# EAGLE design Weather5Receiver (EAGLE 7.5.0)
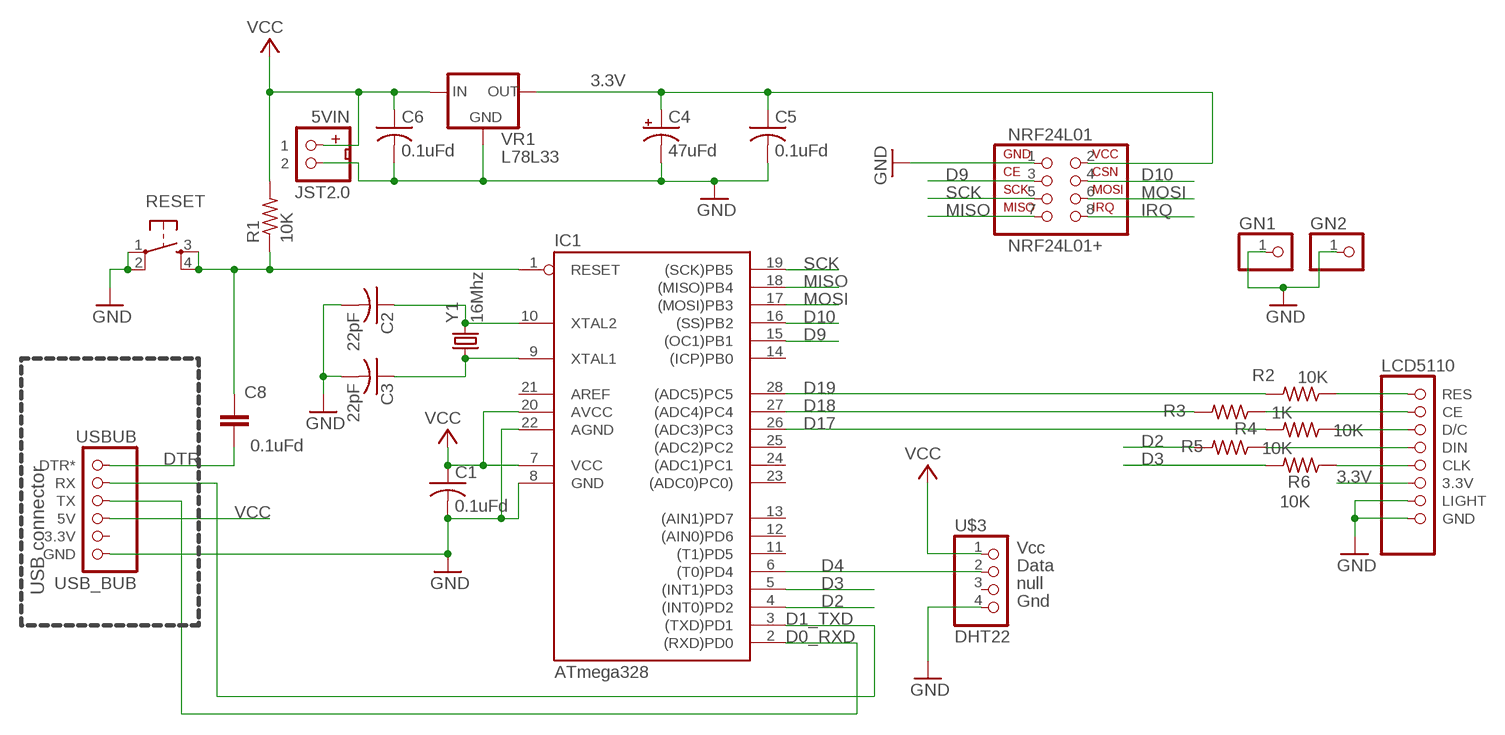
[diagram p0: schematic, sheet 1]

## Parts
5VIN  JST2.0  [JST2.0]
C1  0.1uFd  C-US050-025X075  [C050-025X075]
C2  22pF  C-US025-025X050  [C025-025X050]
C3  22pF  C-US025-025X050  [C025-025X050]
C4  47uFd  CPOL-USE2,5-6E  [E2,5-6E]
C5  0.1uFd  C-US025-025X050  [C025-025X050]
C6  0.1uFd  C-US025-025X050  [C025-025X050]
C8  0.1uFd  C-EU050-025X075  [C050-025X075]
GN1  PINHD-1X1  [1X01]
GN2  PINHD-1X1  [1X01]
IC1  ATmega328  AT90S4433P  [DIL28-3]
LCD5110  LCD5110_1TOP  [LCD5110T1]
NRF24L01  NRF24L01+  [NRF24L01+]
R1  10K  R-US_0207/2V  [0207/2V]
R2  10K  R-US_0207/5V  [0207/5V]
R3  1K  R-US_0207/5V  [0207/5V]
R4  10K  R-US_0207/5V  [0207/5V]
R5  10K  R-US_0207/5V  [0207/5V]
R6  10K  R-US_0207/5V  [0207/5V]
RESET  TAC_SWITCHPTH  [TACTILE-PTH]
U$3  DHT22  [1X04]
USBUB  USB_BUB  [USB_BUB]
VR1  L78L33  78LXX  [78LXX]
Y1  16Mhz  CRYSTALHC49US  [HC49US]

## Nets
3.3V: C4.+ C5.1 LCD5110.3.3V NRF24L01.2 VR1.OUT
D0_RXD: IC1.2((RXD)PD0) USBUB.TX
D1_TXD: IC1.3((TXD)PD1) USBUB.RX
D2: IC1.4((INT0)PD2) R5.2
D3: IC1.5((INT1)PD3) R6.2
D4: IC1.6((T0)PD4) U$3.2(DATA)
D9: IC1.15((OC1)PB1) NRF24L01.3
D10: IC1.16((SS)PB2) NRF24L01.4
D17: IC1.26((ADC3)PC3) R4.2
D18: IC1.27((ADC4)PC4) R3.2
D19: IC1.28((ADC5)PC5) R2.2
DTR: C8.1 USBUB.DTR*
GND [power]: 5VIN.2 C1.2 C2.2 C3.2 C4.- C5.2 C6.2 GN1.1 GN2.1 IC1.8(GND) IC1.22(AGND) LCD5110.GND LCD5110.LIGHT NRF24L01.1 RESET.1 RESET.2 U$3.4(GND) USBUB.GND VR1.GND
IRQ: NRF24L01.8
MISO: IC1.18((MISO)PB4) NRF24L01.7
MOSI: IC1.17((MOSI)PB3) NRF24L01.6
N$1: LCD5110.RES R2.1
N$3: LCD5110.CE R3.1
N$5: LCD5110.D/C R4.1
N$6: C3.1 IC1.9(XTAL1) Y1.1
N$7: C2.1 IC1.10(XTAL2) Y1.2
N$8: LCD5110.DIN R5.1
N$9: LCD5110.CLK R6.1
RESET: C8.2 IC1.1(RESET) R1.1 RESET.3 RESET.4
SCK: IC1.19((SCK)PB5) NRF24L01.5
VCC: 5VIN.1 C1.1 C6.1 IC1.7(VCC) IC1.20(AVCC) R1.2 U$3.1(VCC) USBUB.5V VR1.IN
Unconnected: IC1.11((T1)PD5) IC1.12((AIN0)PD6) IC1.13((AIN1)PD7) IC1.14((ICP)PB0) IC1.21(AREF) IC1.23((ADC0)PC0)) IC1.24((ADC1)PC1) IC1.25((ADC2)PC2) U$3.3(NULL) USBUB.3.3V

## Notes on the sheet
- USB connector

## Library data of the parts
5VIN = MTS_Custom:JST2.0: JST 2.0 2 pin connector 2mm spacing
C1-C3 C5 C6 = MTS:C-US: CAPACITOR, American symbol
C4 = rcl:CPOL-US: POLARIZED CAPACITOR, American symbol
C8 = my-rcl:C-EU: CAPACITOR, European symbol
GN1 GN2 = pinhead:PINHD-1X1: PIN HEADER
IC1 = atmel:AT90S4433: MICROCONTROLLER 4 Kbytes FLASH 128 bytes SRAM 256 bytes EEPROM UART 6-channel 10 bit ADC
LCD5110 = MTS_Custom:LCD5110_1
NRF24L01 = MTS_Custom:NRF24L01+: 2.4GHz Transceiver
R1-R6 = MTS:R-US_: RESISTOR, American symbol
RESET = SparkFun:TAC_SWITCH: Momentary Switch Button commonly used for reset or general input. Spark Fun Electronics SKU : COM-00097
U$3 = MTS_Custom:DHT22: This is a Temperature RH sensor. AKA AMM2303
USBUB = MTS:USB_BUB
VR1 = v-reg:78LXX: VOLTAGE REGULATOR
Y1 = MTS:CRYSTAL: Crystals

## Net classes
0 default: width 0.4 mm, clearance 0.3 mm
1 power: width 0.6 mm, clearance 0.3 mm

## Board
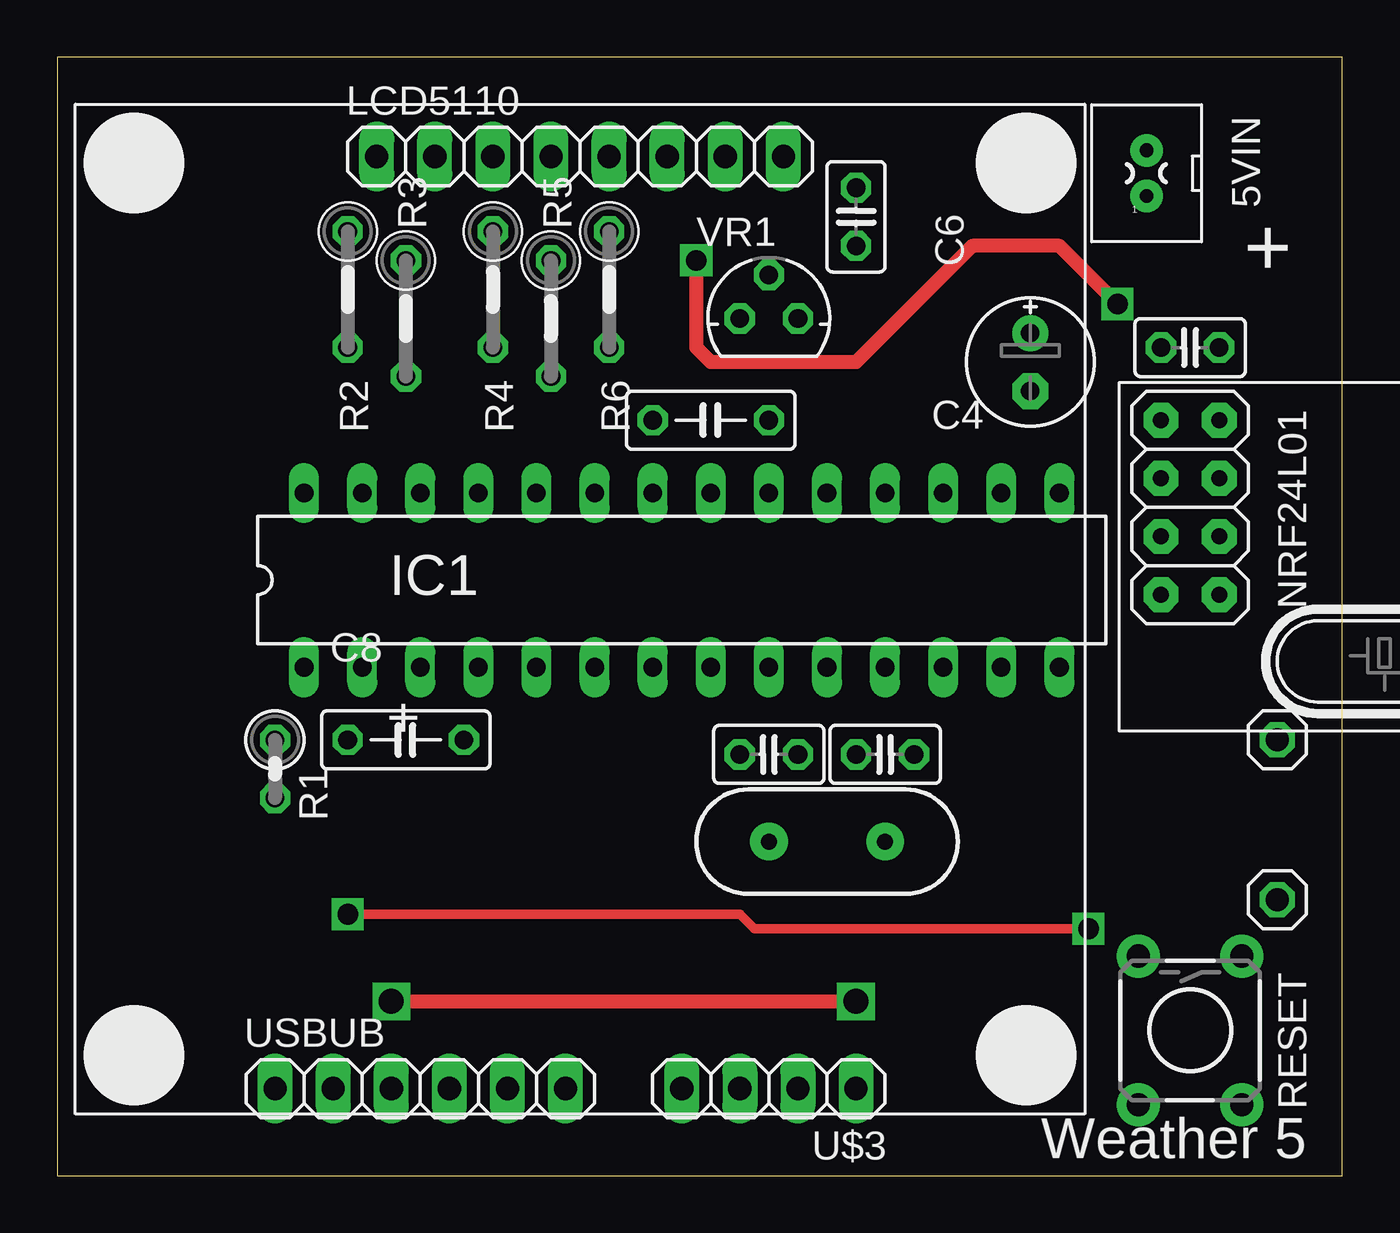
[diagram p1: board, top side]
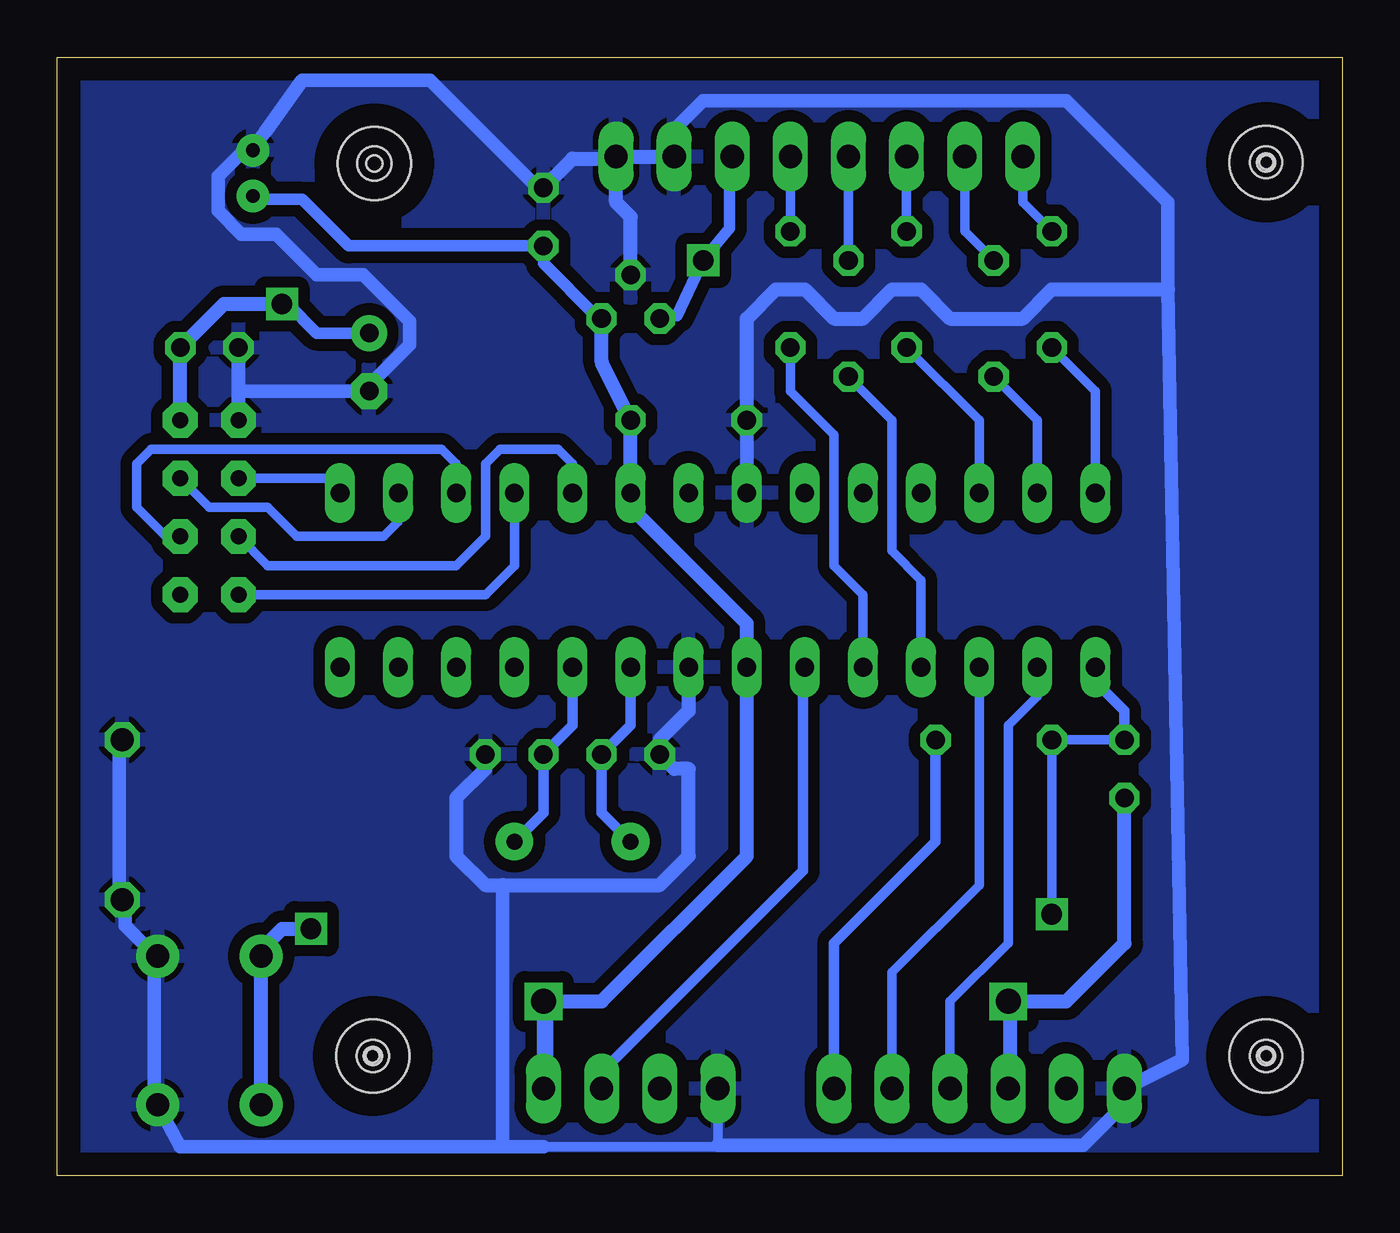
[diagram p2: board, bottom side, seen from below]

Size 56.19 x 48.88 mm. Coordinates in mm from the lower left corner, seen from the top.
Outline: 0,0 56.19,0 56.19,48.88 0,48.88 0,0
Copper layers (1*16): Top 0.035mm / dielectric 1.5mm / Bottom 0.035mm
Design rules "NewMTS": minimum track width 20mil, minimum drill 24mil, track to track 20mil, track to pad 20mil, pad to pad 8mil, via to via 8mil, smd to smd 8mil, copper to edge 40mil, drill to drill 8mil, minimum pad ring 10mil, minimum via ring 10mil, stop-mask expansion 4mil, vias tented up to drill 0mil, thermal gap 10mil
Holes 3.2 mm at 42.32,44.23 42.39,5.24 3.33,5.24 3.33,44.29
Holes 1.5 mm at 42.32,44.23
Holes 0.7 mm at 42.32,44.23
Holes 1.4 mm at 42.39,5.24 3.33,5.24 3.33,44.29
Holes 0.8 mm at 42.39,5.24 3.33,5.24 3.33,44.29
Holes 0.6 mm at 42.39,5.24 3.33,5.24 3.33,44.29

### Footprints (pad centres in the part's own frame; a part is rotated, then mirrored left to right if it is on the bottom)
JST2.0 = drill 0.6 pad 1.422: 1 0,-1; 2 0,1
C050-025X075 = drill 0.813 octagon: 1 -2.54,0; 2 2.54,0
C025-025X050 = drill 0.813 octagon: 1 -1.27,0; 2 1.27,0
E2,5-6E = drill 0.813 pad 1.575: + -1.27,0 | drill 0.813 pad 1.575 octagon: - 1.27,0
1X01 = drill 1.016 octagon: 1 0,0
DIL28-3 = drill 0.813 long: 1 -16.51,-3.81; 2 -13.97,-3.81; 3 -11.43,-3.81; 4 -8.89,-3.81; 5 -6.35,-3.81; 6 -3.81,-3.81; 7 -1.27,-3.81; 8 1.27,-3.81; 9 3.81,-3.81; 10 6.35,-3.81; 11 8.89,-3.81; 12 11.43,-3.81; 13 13.97,-3.81; 14 16.51,-3.81; 15 16.51,3.81; 16 13.97,3.81; 17 11.43,3.81; 18 8.89,3.81; 19 6.35,3.81; 20 3.81,3.81; 21 1.27,3.81; 22 -1.27,3.81; 23 -3.81,3.81; 24 -6.35,3.81; 25 -8.89,3.81; 26 -11.43,3.81; 27 -13.97,3.81; 28 -16.51,3.81
LCD5110T1 = drill 1.016 long: 3.3V 3.81,19.78; CE -6.35,19.78; CLK 1.27,19.78; D/C -3.81,19.78; DIN -1.27,19.78; GND 8.89,19.78; LIGHT 6.35,19.78; RES -8.89,19.78
NRF24L01+ = drill 0.7 pad 1.524 octagon: 1 -5.08,-12.7; 2 -5.08,-10.16; 3 -2.54,-12.7; 4 -2.54,-10.16; 5 0,-12.7; 6 0,-10.16; 7 2.54,-12.7; 8 2.54,-10.16
0207/2V = drill 0.813 octagon: 1 -1.27,0; 2 1.27,0
0207/5V = drill 0.813 octagon: 1 -2.54,0; 2 2.54,0
TACTILE-PTH = drill 1.016 pad 1.88: 1 -3.251,2.261; 2 3.251,2.261; 3 -3.251,-2.261; 4 3.251,-2.261
1X04 = drill 1.016 long: 1 -3.81,0; 2 -1.27,0; 3 1.27,0; 4 3.81,0
USB_BUB = drill 1.016 long: 3.3V -3.81,0; 5V -1.27,0; DTR* 6.35,0; GND -6.35,0; RX 3.81,0; TX 1.27,0
78LXX = drill 0.813 octagon: GND 0,1.905; IN 1.27,0; OUT -1.27,0
HC49US = drill 0.7 pad 1.651: 1 -2.54,0; 2 2.54,0

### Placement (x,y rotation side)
5VIN  47.62,43.81 0 top
C1  28.57,33.02 180 top
C2  36.2,18.41 0 top
C3  31.11,18.41 180 top
C4  42.55,35.56 270 top
C5  49.53,36.2 180 top
C6  34.92,41.91 90 top
C8  15.24,19.05 180 top
GN1  53.34,19.05 0 top
GN2  53.34,12.06 0 top
IC1  27.3,26.04 0 top
LCD5110  22.86,24.77 0 top
NRF24L01  60.96,27.94 270 top
R1  9.53,17.78 270 top
R2  12.7,38.73 270 top
R3  15.24,37.47 270 top
R4  19.05,38.73 270 top
R5  21.59,37.47 270 top
R6  24.13,38.73 270 top
RESET  49.53,6.35 270 top
U$3  31.11,3.81 180 top
USBUB  15.88,3.81 0 top
VR1  31.11,37.47 0 top
Y1  33.66,14.61 0 top

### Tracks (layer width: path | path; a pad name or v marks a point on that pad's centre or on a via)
3.3V  (via drill 0.9)
  Top 0.61: v46.35,38.1 43.81,40.64 40.01,40.64 34.92,35.56 28.57,35.56 27.94,36.2 v27.94,40.01
  Bottom 0.508: VR1.OUT 29.84,37.59 29.08,37.59 v27.94,40.01 26.8,41.4 26.8,44.45 LCD5110.3.3V | C4.+ 44.83,36.83 46.1,38.1 v46.35,38.1
  Bottom 0.61: NRF24L01.2 C5.1 48.9,38.1 v46.35,38.1
D0_RXD
  Bottom 0.406: IC1.2 13.34,20.95 14.61,19.68 14.61,10.16 17.14,7.62 USBUB.TX
D1_TXD
  Bottom 0.406: IC1.3 15.88,12.7 19.68,8.89 USBUB.RX
D2
  Bottom 0.406: IC1.4 18.41,26.04 19.68,27.3 19.68,33.02 R5.2
D3
  Bottom 0.406: IC1.5 20.95,25.4 22.23,26.67 22.23,32.38 24.13,34.29 R6.2
D4
  Bottom 0.457: U$3.2 32.38,4.53 23.58,13.34 23.58,22.14 IC1.6
D9
  Bottom 0.406: IC1.15 44.45,30.48 NRF24L01.3
D10
  Bottom 0.406: IC1.16 41.27,28.57 41.91,27.94 45.72,27.94 46.99,29.21 49.53,29.21 NRF24L01.4
D17
  Bottom 0.406: IC1.26 15.88,33.02 R4.2
D18
  Bottom 0.406: IC1.27 13.34,33.02 R3.2
D19
  Bottom 0.406: IC1.28 10.79,34.29 R2.2
DTR
  Bottom 0.457: C8.1 17.78,14.61 22.23,10.16 USBUB.DTR*
GND
  Bottom 0.406: 34.92,1.27 27.3,1.27 27.3,1.33 U$3.4
  Bottom 0.6: C1.2 IC1.22 | 36.7,1.27 50.8,1.27 RESET.2 51.94,3.3 51.94,9.4 RESET.1 51.94,9.65 53.21,10.92 53.21,11.94 GN2.1 53.47,12.19 53.47,19.05 GN1.1 | 36.7,1.27 34.92,1.27 | 27.32,1.33 27.3,1.33 11.32,1.33 9.72,2.93 9.72,3.73 USBUB.GND 6.99,5.08 7.62,38.73 7.62,42.55 12.06,46.99 27.94,46.99 29.08,45.85 29.08,44.45 LCD5110.LIGHT 29.34,44.45 | 48.26,34.29 C4.- 42.55,34.54 40.77,36.32 40.77,37.34 42.8,39.37 44.83,39.37 46.61,41.15 48.13,41.15 49.15,42.16 49.15,43.69 47.88,44.96 5VIN.2 47.62,44.96 47.12,45.59 45.47,47.88 39.88,47.88 35.18,43.18 C6.2 | 36.7,1.27 36.7,12.7
  Bottom 0.61: NRF24L01.1 48.26,34.29 C5.2 | IC1.8 28.57,20.32 29.84,19.05 C3.2 29.21,17.78 28.57,17.78 28.57,13.97 29.84,12.7 36.7,12.7 37.47,12.7 38.73,13.97 38.73,16.51 37.47,17.78 C2.2 | C6.2 33.66,44.45 31.84,44.45 LCD5110.GND | LCD5110.GND LCD5110.LIGHT 29.3,44.55 | VR1.GND 31.11,41.91 31.75,42.55 LCD5110.GND | C1.2 26.04,37.47 24.77,38.73 23.5,38.73 22.23,37.47 20.95,37.47 19.68,38.73 18.41,38.73 17.14,37.47 13.97,37.47 12.7,38.73 7.62,38.73
  pour Bottom: 0,0 0,48.9 56.52,48.9 56.52,0
MISO
  Bottom 0.406: NRF24L01.7 37.47,25.4 36.2,26.67 IC1.18
MOSI
  Bottom 0.406: NRF24L01.6 51.44,27.94 52.7,29.21 52.7,31.11 52.07,31.75 39.37,31.75 38.73,31.11 IC1.17
N$1
  Bottom 0.406: LCD5110.RES 13.97,42.55 R2.1
N$3
  Bottom 0.406: LCD5110.CE 16.51,41.27 R3.1
N$5
  Bottom 0.406: R4.1 LCD5110.D/C
N$6
  Bottom 0.457: Y1.1 32.38,15.88 C3.1 31.11,19.68 IC1.9
N$7
  Bottom 0.457: Y1.2 34.92,15.88 C2.1 33.66,19.68 IC1.10
N$8
  Bottom 0.406: R5.1 LCD5110.DIN
N$9
  Bottom 0.406: R6.1 LCD5110.CLK
RESET  (via drill 0.9)
  Top 0.406: v45.09,10.79 30.48,10.79 29.84,11.43 v12.7,11.43
  Bottom 0.406: R1.1 C8.2 v12.7,11.43
  Bottom 0.457: R1.1 9.53,20.32 10.79,21.59 IC1.1
  Bottom 0.61: RESET.4 RESET.3 47.27,9.88 46.35,10.79 v45.09,10.79
SCK
  Bottom 0.406: IC1.19 33.66,31.11 34.29,31.75 36.83,31.75 37.47,31.11 37.47,27.94 38.73,26.67 46.99,26.67 NRF24L01.5
VCC  (via drill 1.1)
  Top 0.61: v14.61,7.62 v34.92,7.62
  Bottom 0.457: 14.52,4.53 14.52,4 USBUB.5V | 34.78,4.53 34.78,4 U$3.1
  Bottom 0.508: VR1.IN 32.64,37.59 34.92,39.88 C6.1 43.43,40.64 45.47,42.67 47.62,42.67 5VIN.1
  Bottom 0.61: VR1.IN 32.38,35.56 C1.1 IC1.20 31.11,29.21 26.04,24.13 IC1.7 26.04,13.97 32.38,7.62 v34.92,7.62 | v34.92,7.62 U$3.1 | 14.52,4.53 14.52,7.53 v14.61,7.62 12.06,7.62 9.53,10.16 R1.2 | 34.78,4.53 34.78,7.48 v34.92,7.62

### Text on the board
tPlace: + | Weather 5
tNames: +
